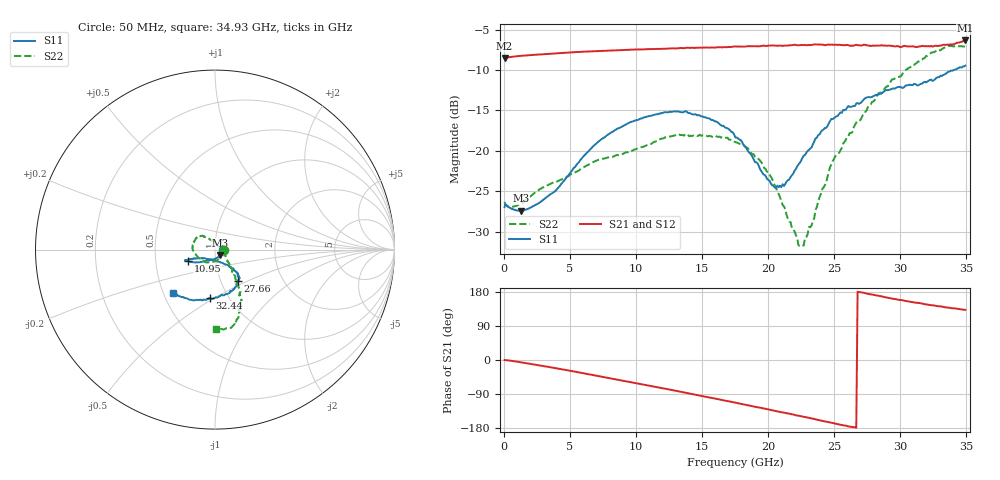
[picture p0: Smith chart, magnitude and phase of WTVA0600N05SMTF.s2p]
! 50 ohm 2-Port S-parameters measured by Modelithics Inc support@modelithics.com  Tampa, FL USA 813-866-6335 (February 2024)
! Smiths Interconnect,  6dB P/N: WTVA0600N05SMTF, Temperature: -25 C
! Board: 10 mil Rogers 4350B, Mounting Pad Dimensions: Length: 15 mils, Width: 25 mils, Gap: 40 mils.
# Hz S RI R 50
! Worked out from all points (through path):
!   352 points, 50 MHz to 34.93 GHz, reference 50 ohm
!   highest |S21| = -6.34 dB at 34.93 GHz (marker M1); lowest = -8.5 dB at 50 MHz (marker M2)
!   group delay of S21, straight-line fit = 19 ps
!   lowest |S11| = -27.4 dB at 1.294 GHz (marker M3), VSWR 1.09, Z = 53 - j3.22 ohm
!   |S11| at or under -10 dB: start of sweep to 34.05 GHz
!   |S22| runs from -31.8 to -7.0 dB; largest |S21 - S12| = 0.005
!   S11 on the Smith chart (normalised r, x): 50 MHz: 1.09, -0.00; 10.95 GHz: 0.73, -0.10; 27.66 GHz: 1.21, -0.44; 32.44 GHz: 0.82, -0.47; 34.93 GHz: 0.56, -0.31
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5e7  0.0449 -0.00163  0.3753 -3.32e-05  0.375 -0.00025  0.0483 -0.00158
3.99e8  0.0423 -0.0144  0.3794 -0.0087  0.3791 -0.00883  0.0423 -0.0157
1.2945e9  0.0299 -0.0303  0.3849 -0.0413  0.3844 -0.0414  0.0317 -0.0348
3.8815e9  -0.0129 -0.055  0.3732 -0.1459  0.3725 -0.1462  0.00286 -0.0641
5.8715e9  -0.0607 -0.0659  0.3402 -0.2286  0.3396 -0.2287  -0.031 -0.0711
8.359e9  -0.1132 -0.0714  0.2685 -0.3206  0.2674 -0.3209  -0.0691 -0.0621
1.0946e10  -0.1509 -0.0637  0.164 -0.3928  0.1624 -0.3929  -0.1053 -0.0297
1.1742e10  -0.1584 -0.0614  0.1269 -0.4081  0.1257 -0.408  -0.1161 -0.0168
1.48265e10  -0.1552 -0.0583  -0.0297 -0.4339  -0.0305 -0.4333  -0.1182 0.0432
1.7513e10  -0.1106 -0.0489  -0.1718 -0.4072  -0.1728 -0.4062  -0.0859 0.0741
1.9304e10  -0.0641 -0.0479  -0.2558 -0.3616  -0.2569 -0.3603  -0.0545 0.0699
2.05975e10  -0.0177 -0.0565  -0.3157 -0.3165  -0.3166 -0.3149  -0.0241 0.0543
2.11945e10  -0.000502 -0.0606  -0.3372 -0.2941  -0.3378 -0.2928  -0.0104 0.0441
2.2289e10  0.0373 -0.0734  -0.3773 -0.245  -0.3779 -0.2433  0.0162 0.0205
2.2687e10  0.049 -0.0795  -0.3903 -0.226  -0.3905 -0.2246  0.0218 0.014
2.3085e10  0.0585 -0.0829  -0.4019 -0.2061  -0.4019 -0.205  0.0337 0.00404
2.33835e10  0.0696 -0.0849  -0.4101 -0.1933  -0.4102 -0.1921  0.0366 -0.00502
2.4876e10  0.1056 -0.1164  -0.4403 -0.1076  -0.4403 -0.1061  0.0673 -0.0538
2.7662e10  0.1274 -0.173  -0.4453 0.0493  -0.4445 0.0514  0.1125 -0.1562
2.91545e10  0.1123 -0.2102  -0.4302 0.1252  -0.4291 0.1271  0.1384 -0.2195
3.2438e10  -0.0298 -0.269  -0.3582 0.2579  -0.3563 0.2599  0.1213 -0.3882
3.49255e10  -0.2343 -0.2414  -0.3233 0.3572  -0.3199 0.3596  0.00436 -0.4414
